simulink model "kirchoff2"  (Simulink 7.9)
settings: Solver=ode23s  StartTime=0.0  StopTime=1  RelTol=1e-3
libraries: fl_lib x8, nesl_utility x5, powerlib x1

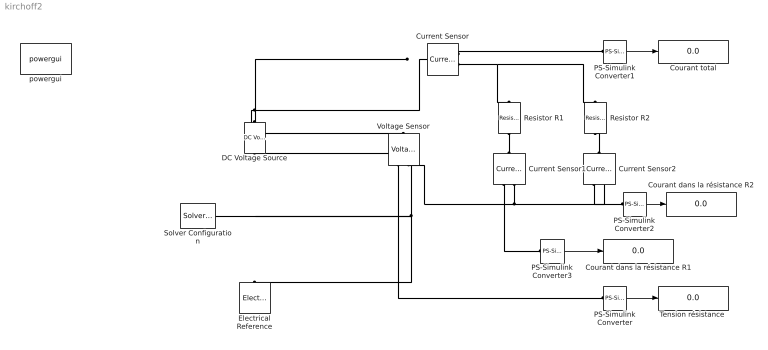
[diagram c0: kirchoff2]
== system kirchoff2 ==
  Courant dans la résistance R1 : Display
  Courant dans la résistance R2 : Display
  Courant total : Display
  Current Sensor : fl_lib/Electrical/Electrical Sensors/Current Sensor  i1_Log=off  v1_Log=off  LocalVarNames=|i1|v1  LocalVarDescs=|i1|v1  LocalVarLogging=[0 0]
  Current Sensor1 : fl_lib/Electrical/Electrical Sensors/Current Sensor  i1_Log=off  v1_Log=off  LocalVarNames=|i1|v1  LocalVarDescs=|i1|v1  LocalVarLogging=[0 0]
  Current Sensor2 : fl_lib/Electrical/Electrical Sensors/Current Sensor  i1_Log=off  v1_Log=off  LocalVarNames=|i1|v1  LocalVarDescs=|i1|v1  LocalVarLogging=[0 0]
  DC Voltage Source : fl_lib/Electrical/Electrical Sources/DC Voltage Source  v0=10 V  i_Log=off  v_Log=off  LocalVarNames=|i|v  LocalVarDescs=|i|v  LocalVarLogging=[0 0]
  Electrical Reference : fl_lib/Electrical/Electrical Elements/Electrical Reference  i_Log=off  LocalVarNames=|i  LocalVarDescs=|i  LocalVarLogging=0
  PS-Simulink Converter : nesl_utility/PS-Simulink Converter  PhysicalDomain=network_engine_domain  LeftPortType=input  RightPortType=output  SubClassName=ps_output  Unit=V  AffineConversion=off
  PS-Simulink Converter1 : nesl_utility/PS-Simulink Converter  PhysicalDomain=network_engine_domain  LeftPortType=input  RightPortType=output  SubClassName=ps_output  Unit=A  AffineConversion=off
  PS-Simulink Converter2 : nesl_utility/PS-Simulink Converter  PhysicalDomain=network_engine_domain  LeftPortType=input  RightPortType=output  SubClassName=ps_output  Unit=A  AffineConversion=off
  PS-Simulink Converter3 : nesl_utility/PS-Simulink Converter  PhysicalDomain=network_engine_domain  LeftPortType=input  RightPortType=output  SubClassName=ps_output  Unit=A  AffineConversion=off
  Resistor R1 : fl_lib/Electrical/Electrical Elements/Resistor  R=50 Ohm  i_Log=off  v_Log=off  LocalVarNames=|i|v  LocalVarDescs=|i|v  LocalVarLogging=[0 0]
  Resistor R2 : fl_lib/Electrical/Electrical Elements/Resistor  R=50 Ohm  i_Log=off  v_Log=off  LocalVarNames=|i|v  LocalVarDescs=|i|v  LocalVarLogging=[0 0]
  Solver Configuration : nesl_utility/Solver Configuration  PhysicalDomain=network_engine_domain  LeftPortType=input  RightPortType=generic  SubClassName=solver  UseCustomDae=off  DoDC=off  ResidualTolerance=1e-9  UseLocalSolver=off  LocalSolverChoice=NE_BACKWARD_EULER_ADVANCER  LocalSolverSampleTime=.001  DoFixedCost=off  MaxNonlinIter=3  MaxModeIter=2  LinearAlgebra=Sparse  Accelerate=off  Profile=off  UseLocalSampling=off  DelaysMemoryBudget=1024
  "Tension résistance " : Display
  Voltage Sensor : fl_lib/Electrical/Electrical Sensors/Voltage Sensor  i1_Log=off  v1_Log=off  LocalVarNames=|i1|v1  LocalVarDescs=|i1|v1  LocalVarLogging=[0 0]
  powergui : powerlib/powergui  Priority=1  SimulationMode=Continuous  SolverType=Tustin  SampleTime=50e-6  frequency=60  SPID=off  DisableSnubberDevices=off  DisableRonSwitches=off  DisableVfSwitches=off  SwTol=0  Interpol=off  DisplayEquations=off  FunctionMessages=off  frequencyindice=17  Pbase=100e6  ErrMax=1e-4  Iterations=50  UnitsV=V  UnitsW=W  echomessages=off  HookPort=off  EnableUseOfTLC=off  x0status=blocks  RestoreLinks=warning  ResistiveCurrentMeasurement=off  Ylog=off  Xlog=on  ShowGrid=off  save=off  variable=ZData  ZoomFFT=off  StartTime=0.0  cycles=1  DisplayStyle=1  FreqAxis=off  MaxFrequency=1000  frequencyindicesteady=1  display=off  methode=off
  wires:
  PS-Simulink Converter1/1 -> Courant total/1
  PS-Simulink Converter/1 -> "Tension résistance "/1
  PS-Simulink Converter2/1 -> Courant dans la résistance R2/1
  PS-Simulink Converter3/1 -> Courant dans la résistance R1/1
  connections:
  Current Sensor1/RConn2 -- Electrical Reference/LConn1 -- DC Voltage Source/RConn1 -- Solver Configuration/RConn1 -- Voltage Sensor/RConn2 -- Current Sensor2/RConn2
  DC Voltage Source/LConn1 -- Voltage Sensor/LConn1 -- Current Sensor/LConn1
  Current Sensor/RConn1 -- PS-Simulink Converter1/LConn1
  Current Sensor/RConn2 -- Resistor R1/LConn1 -- Resistor R2/LConn1
  Voltage Sensor/RConn1 -- PS-Simulink Converter/LConn1
  Resistor R1/RConn1 -- Current Sensor1/LConn1
  Resistor R2/RConn1 -- Current Sensor2/LConn1
  Current Sensor2/RConn1 -- PS-Simulink Converter2/LConn1
  Current Sensor1/RConn1 -- PS-Simulink Converter3/LConn1
